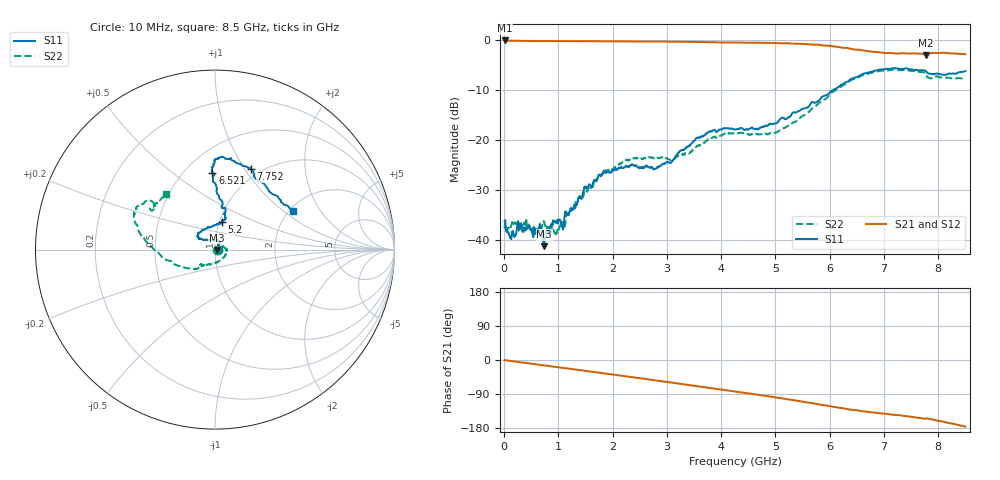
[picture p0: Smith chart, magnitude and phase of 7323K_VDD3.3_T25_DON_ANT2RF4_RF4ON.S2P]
!Agilent Technologies,E5071C,MY46417908,A.11.23
!Date: Mon Jan 18 17:06:38 2021
!Data & Calibration Information:
!Freq	S11:SOLT2(ON)	S21:SOLT2(ON)	S12:SOLT2(ON)	S22:SOLT2(ON)
!PortZ  Port1:50+j0  Port2:50+j0
!Above PortZ is port z conversion or system Z0 setting when saving the data.
!When reading, reference impedance value at option line is always used.
# Hz S dB R 50
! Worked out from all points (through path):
!   1601 points, 10 MHz to 8.5 GHz, reference 50 ohm
!   highest |S21| = -0.16 dB at 10 MHz (marker M1); lowest = -3.0 dB at 7.778 GHz (marker M2)
!   group delay of S21, straight-line fit = 56.7 ps
!   lowest |S11| = -41.3 dB at 737 MHz (marker M3), VSWR 1.02, Z = 50.8 - j0.165 ohm
!   |S11| at or under -10 dB: start of sweep to 6.078 GHz
!   |S22| runs from -38.9 to -6.0 dB; largest |S21 - S12| = 0.0079
!   S11 on the Smith chart (normalised r, x): 10 MHz: 1.03, -0.00; 5.2 GHz: 1.03, +0.33; 6.521 GHz: 0.67, +0.71; 7.752 GHz: 0.90, +1.07; 8.5 GHz: 2.09, +1.18
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1e7  -36.28 -1.3  -0.16 -0.3  -0.16 -0.3  -37.76 -11.9
1.002062e8  -39.14 -13.2  -0.20 -2.1  -0.20 -2.1  -37.57 -14.4
2.85925e8  -38.01 -17.8  -0.23 -5.7  -0.24 -5.7  -37.30 -18.3
6.573625e8  -36.86 -19.0  -0.26 -12.7  -0.26 -12.7  -37.43 -26.4
7.369562e8  -41.33 -10.9  -0.27 -14.2  -0.27 -14.2  -36.38 -20.2
9.704312e8  -36.37 15.0  -0.28 -18.6  -0.28 -18.6  -38.74 -0.2
1.07125e9  -37.42 18.5  -0.28 -20.5  -0.29 -20.5  -36.73 -5.4
1.426769e9  -31.86 49.4  -0.30 -27.3  -0.30 -27.3  -31.60 21.4
1.851269e9  -26.30 60.1  -0.32 -35.4  -0.33 -35.4  -26.34 19.9
2.365975e9  -25.03 70.4  -0.35 -45.4  -0.35 -45.4  -23.81 0.3
2.843538e9  -25.55 102.4  -0.37 -54.9  -0.37 -54.8  -23.72 -34.6
3.103544e9  -24.29 124.7  -0.39 -60.0  -0.39 -60.0  -23.94 -58.8
3.761519e9  -18.57 143.4  -0.50 -73.2  -0.50 -73.2  -19.88 -120.9
4.255e9  -17.94 128.2  -0.56 -82.9  -0.57 -82.9  -18.71 -133.8
5.199512e9  -15.88 76.2  -0.69 -103.1  -0.70 -103.1  -17.44 -131.7
5.671769e9  -12.51 76.1  -1.00 -113.9  -0.98 -114.0  -13.81 -151.0
6.520769e9  -7.36 91.9  -2.00 -133.1  -2.03 -133.1  -7.57 169.0
7.088538e9  -5.84 88.1  -2.64 -142.7  -2.67 -142.9  -6.11 155.8
7.751819e9  -6.18 65.9  -2.97 -155.1  -2.99 -155.0  -6.67 143.7
7.77835e9  -6.35 63.5  -3.04 -154.6  -3.06 -154.6  -7.14 142.6
7.9057e9  -6.90 57.9  -2.63 -157.2  -2.65 -157.2  -7.57 148.6
8.5e9  -6.28 26.3  -2.91 -175.8  -2.98 -176.0  -7.65 131.3
